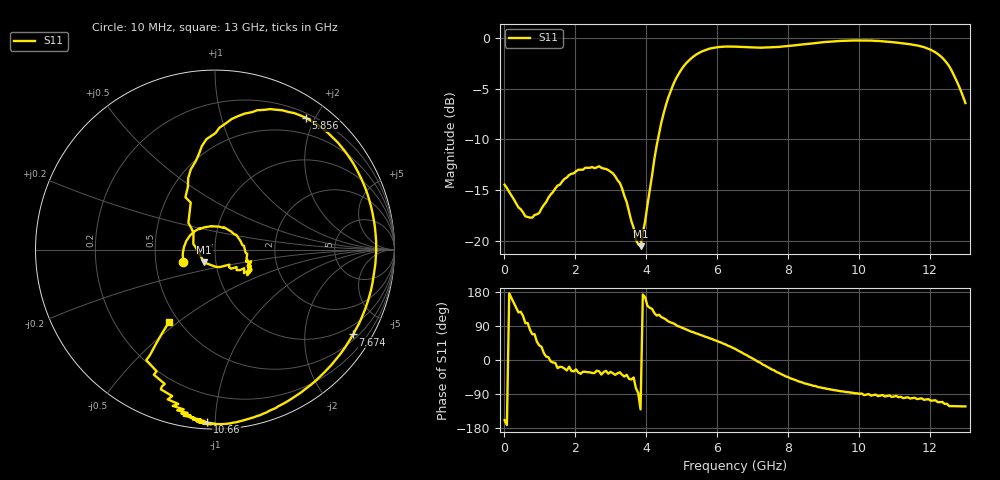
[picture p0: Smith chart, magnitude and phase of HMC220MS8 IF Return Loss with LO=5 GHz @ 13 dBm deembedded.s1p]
!Hittite Microwave Corporation
!12 Elizabeth Drive
!Chelmsford, MA 01824
!Tel: 978-250-3343
!Fax: 978-250-3373
!Device: HMC220MS8, 5-12 GHz, GaAS MMIC SMT Double-Balanced Mixer in 8-lead MSOP package
!Misc: IF Return Loss, LO = 5 GHz @ 13dBm, Room
# MHZ S MA R 50
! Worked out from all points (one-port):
!   201 points, 10 MHz to 13 GHz, reference 50 ohm
!   lowest |S11| = -20.5 dB at 3.842 GHz (marker M1), VSWR 1.21, Z = 43.8 - j6.35 ohm
!   |S11| at or under -10 dB: start of sweep to 4.332 GHz
!   S11 on the Smith chart (normalised r, x): 10 MHz: 0.69, -0.10; 5.856 GHz: 0.26, +1.88; 7.674 GHz: 0.67, -3.42; 10.66 GHz: 0.04, -0.96; 13 GHz: 0.44, -0.46
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10  0.189 -159.0
334.75  0.153 138.2
594.55  0.132 97.4
1114.15  0.15 18.7
1633.75  0.196 -18.8
2672.95  0.233 -29.8
3257.5  0.193 -32.5
3647.2  0.116 -46.1
3842.05  0.094 -130.2
4426.6  0.382 113.2
4881.25  0.649 89.7
5335.9  0.811 73.2
5855.5  0.892 55.4
6505  0.907 29.6
7089.55  0.898 -0.7
7674.1  0.903 -31.6
8128.75  0.918 -50.4
8843.2  0.948 -71.5
9752.5  0.972 -85.8
10077.25  0.973 -88.3
10142.2  0.973 -92.7
10661.8  0.963 -92.5
11051.5  0.95 -94.7
11246.35  0.942 -100.6
11376.25  0.935 -98.3
12155.65  0.85 -106.3
12545.35  0.725 -121.9
13000  0.478 -122.4
